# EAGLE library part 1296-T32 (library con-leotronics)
1.27mm SINGLE ROW FEMALE SOCKET Source: http://www.leotronics.co.uk/Conexcon/Data%20Sheets/sec.%20A/1296ing.pdf
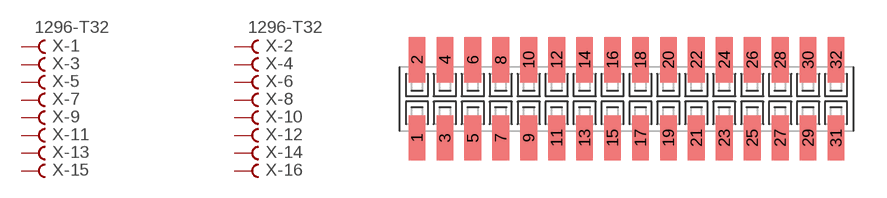
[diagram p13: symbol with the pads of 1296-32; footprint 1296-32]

Designator prefix X; gates -1=FVAL -2=FVAL -3=F -4=F -5=F -6=F -7=F -8=F -9=F -10=F -11=F -12=F -13=F -14=F -15=F -16=F -17=F -18=F -19=F -20=F -21=F -22=F -23=F -24=F -25=F -26=F -27=F -28=F -29=F -30=F -31=F -32=F

## 1296-T32 (OC_FARNELL: unknown; OC_NEWARK: unknown)  [1296-32]
1  -1:B  pas
2  -2:B  pas
3  -3:B  pas
4  -4:B  pas
5  -5:B  pas
6  -6:B  pas
7  -7:B  pas
8  -8:B  pas
9  -9:B  pas
10  -10:B  pas
11  -11:B  pas
12  -12:B  pas
13  -13:B  pas
14  -14:B  pas
15  -15:B  pas
16  -16:B  pas
17  -17:B  pas
18  -18:B  pas
19  -19:B  pas
20  -20:B  pas
21  -21:B  pas
22  -22:B  pas
23  -23:B  pas
24  -24:B  pas
25  -25:B  pas
26  -26:B  pas
27  -27:B  pas
28  -28:B  pas
29  -29:B  pas
30  -30:B  pas
31  -31:B  pas
32  -32:B  pas

## Footprint 1296-32 (pad centres in mm)
1.27mm SINGLE ROW FEMALE SOCKET Source: http://www.leotronics.co.uk/Conexcon/Data%20Sheets/sec.%20A/1296ing.pdf
smd 0.76 x 2.05: 1 -9.525,-1.78; 2 -9.525,1.78; 3 -8.255,-1.78; 4 -8.255,1.78; 5 -6.985,-1.78; 6 -6.985,1.78; 7 -5.715,-1.78; 8 -5.715,1.78; 9 -4.445,-1.78; 10 -4.445,1.78; 11 -3.175,-1.78; 12 -3.175,1.78; 13 -1.905,-1.78; 14 -1.905,1.78; 15 -0.635,-1.78; 16 -0.635,1.78; 17 0.635,-1.78; 18 0.635,1.78; 19 1.905,-1.78; 20 1.905,1.78; 21 3.175,-1.78; 22 3.175,1.78; 23 4.445,-1.78; 24 4.445,1.78; 25 5.715,-1.78; 26 5.715,1.78; 27 6.985,-1.78; 28 6.985,1.78; 29 8.255,-1.78; 30 8.255,1.78; 31 9.525,-1.78; 32 9.525,1.78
